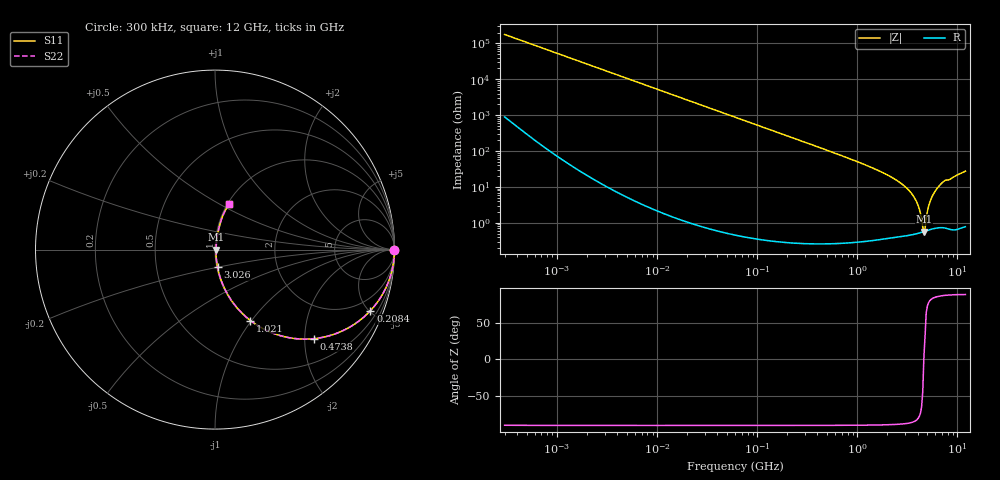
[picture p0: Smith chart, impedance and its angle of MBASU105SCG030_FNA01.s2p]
! MBASU105SCG030_FNA01  S-PARAMETER MODEL  ( Standard Model )
! Model Generated by TAIYO YUDEN Corporation (http://www.ty-top.com)
! Version 1.0
! TAIYO YUDEN Control No. 230609
! Copyright(c) 2023 TAIYO YUDEN CO.,LTD. All Rights Reserved.
! Product Description (link to TY-COMPAS)
! https://ds.yuden.co.jp/TYCOMPAS/or/detail?pn=MBASU105SCG030BFNA01&u=M
! Products Name : Multilayer Ceramic Capacitors
! Characteristics :
!  Capacitance : 3 [pF] , Rated Voltage : 50 [V] , TCC : CG / C0G
!  Case Size : 1.0 x 0.5 / 0.039 x 0.02 [mm/inch] , Thickness : 0.5 / 0.02 [mm/inch]
!  (Conditions: Temperature = 25 [degC] , DC Bias Voltage = 0 [V])
! External Node Assignments :
!  1  o---| |---o  2
! GND o---------o GND
! Frequency Range : 0.3MHz  -  12000MHz  [ 401 STEP ]
# MHZ S RI R 50
! Freq[MHz].  S11 Real  S11 Imag  S21 Real  S21 Imag  S12 Real  S12 Imag  S22 Real  S22 Imag
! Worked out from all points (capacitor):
!   401 points, 300 kHz to 12 GHz, reference 50 ohm
!   read as one part in series: C = 3 pF near 316.3 kHz
!   lowest |Z| = 573 mohm at 4.624 GHz (marker M1)
!   series resonance near 4.615 GHz, so ESL is about 400 pH
!   S11 on the Smith chart (normalised r, x): 300 kHz: open; 208.4 MHz: 1.01, -5.08; 473.8 MHz: 1.01, -2.22; 1.021 GHz: 1.01, -0.99; 3.026 GHz: 1.01, -0.20; 12 GHz: 1.02, +0.55
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0.3  1 -0.000565  3.18e-06 0.000565  3.18e-06 0.000565  1 -0.000565
1.769972  1 -0.00334  1.4e-05 0.00334  1.4e-05 0.00334  1 -0.00334
10.44266  0.9996 -0.0197  0.000395 0.0197  0.000395 0.0197  0.9996 -0.0197
60  0.9873 -0.1117  0.0127 0.1117  0.0127 0.1117  0.9873 -0.1117
208.3979  0.8656 -0.3406  0.1344 0.3406  0.1344 0.3406  0.8656 -0.3406
353.9943  0.6891 -0.462  0.3109 0.462  0.3109 0.462  0.6891 -0.462
473.7541  0.551 -0.4962  0.449 0.4962  0.449 0.4962  0.551 -0.4962
1021.415  0.1975 -0.3952  0.8025 0.3952  0.8025 0.3952  0.1975 -0.3952
2088.533  0.0424 -0.1925  0.9576 0.1925  0.9576 0.1925  0.0424 -0.1925
3026.31  0.014 -0.0979  0.986 0.0979  0.986 0.0979  0.014 -0.0979
3454.93  0.00902 -0.0663  0.991 0.0663  0.991 0.0663  0.00902 -0.0663
3841.137  0.00664 -0.0417  0.9934 0.0417  0.9934 0.0417  0.00664 -0.0417
4158.869  0.00574 -0.0234  0.9943 0.0234  0.9943 0.0234  0.00574 -0.0234
4502.883  0.00558 -0.00524  0.9944 0.00524  0.9944 0.00524  0.00558 -0.00524
4623.766  0.00568 0.000404  0.9943 -0.000404  0.9943 -0.000404  0.00568 0.000404
4747.894  0.00583 0.00363  0.9942 -0.00363  0.9942 -0.00363  0.00583 0.00363
4875.354  0.00611 0.012  0.9939 -0.012  0.9939 -0.012  0.00611 0.012
5140.631  0.00702 0.0274  0.993 -0.0274  0.993 -0.0274  0.00702 0.0274
5420.343  0.00847 0.0435  0.9915 -0.0435  0.9915 -0.0435  0.00847 0.0435
6354.153  0.0161 0.0938  0.9839 -0.0938  0.9839 -0.0938  0.0161 0.0938
7448.838  0.0287 0.1446  0.9713 -0.1446  0.9713 -0.1446  0.0287 0.1446
12000  0.0767 0.2522  0.9233 -0.2522  0.9233 -0.2522  0.0767 0.2522
